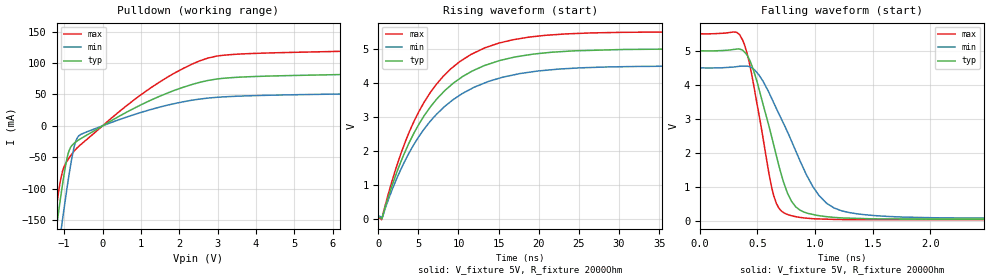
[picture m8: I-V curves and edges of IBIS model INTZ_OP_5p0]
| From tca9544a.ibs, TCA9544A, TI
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|   Model
[Model]   INTZ_OP_5p0
Model_type   Open_drain
Polarity   Non-Inverting
Vmeas = 2.5
Vref = 5
Cref = 1pF
Rref = 2000
|   typ   min   max
C_comp   1.601pF   1.487pF   1.862pF
[Voltage Range]   5   4.5   5.5
[Temperature Range]   27   125   -40
[Pullup Reference]   5   4.5   5.5
[Pulldown Reference]   -0   -0   -0
[Power Clamp Reference]   5   4.5   5.5
[GND Clamp Reference]   -0   -0   -0
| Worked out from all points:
|   slope of the pulldown table from 0 to 0.75 V, typ, clamps not added: 29.2 ohm
|   falling waveform, V_fixture 5V, R_fixture 2000Ohm: 20-80 % time 234ps typ, 368ps min, 171ps max; typ from 5 V to 0.068 V
|   rising waveform, V_fixture 5V, R_fixture 2000Ohm: 20-80 % time 7.63ns typ, 8.08ns min, 7.26ns max; typ from 0.068 V to 5 V
[Pulldown]
|   Voltage   I(typ)   I(min)   I(max)
-5V       -2.025A    -2.08A     -1.991A
-1.61V    -353.8mA   -413.6mA   -316.9mA
-1.25V    -183.9mA   -243.3mA   -148.6mA
-1.085V   -110.6mA   -167.8mA   -83.22mA
-1.025V   -85.9mA    -141.2mA   -68.54mA
-875mV    -39.88mA   -78.44mA   -51.42mA
-740mV    -27.74mA   -33.39mA   -40.24mA
-620mV    -22.36mA   -15.97mA   -32.64mA
1.27V     41.23mA    26.19mA    61.07mA
2.74V     72.2mA     44.16mA    107.9mA
7.435V    84.91mA    53.7mA     123.1mA
9.985V    125mA      83.55mA    179.8mA
[Ramp]
R_load = 2000
|   typ   min   max
dV/dt_r   2.95938/7.62679e-09   2.64368/8.08593e-09   3.26962/7.25871e-09
dV/dt_f   2.9594/2.33624e-10   2.64369/3.68147e-10   3.26964/1.70673e-10
[Falling Waveform]
V_fixture = 5V
V_fixture_min = 4.5V
V_fixture_max = 5.5V
R_fixture = 2000Ohm
C_fixture = 0F
|   Time   V(typ)   V(min)   V(max)
0s        5V         4.5V       5.5V
373.1ps   5.011V     4.551V     5.3V
461.7ps   4.47V      4.474V     4.089V
607.5ps   2.687V     3.719V     1.254V
685.3ps   1.636V     3.156V     389.6mV
830.9ps   430.4mV    2.073V     139.8mV
1.033ns   168.9mV    760.6mV    72.68mV
1.193ns   110.9mV    356.8mV    56.02mV
3.18ns    68.08mV    94.31mV    52mV
100ns     67.67mV    93.83mV    50.6mV
[Rising Waveform]
V_fixture = 5V
V_fixture_min = 4.5V
V_fixture_max = 5.5V
R_fixture = 2000Ohm
C_fixture = 0F
|   Time   V(typ)   V(min)   V(max)
0s        67.67mV    93.83mV    50.6mV
448.6ps   20.09mV    53.71mV    2.403mV
2.057ns   1.211V     1.055V     1.382V
3.952ns   2.295V     1.993V     2.611V
5.662ns   3.018V     2.633V     3.416V
7.167ns   3.495V     3.059V     3.941V
11.54ns   4.332V     3.828V     4.84V
16.68ns   4.748V     4.231V     5.268V
32.43ns   4.991V     4.489V     5.494V
100ns     5V         4.5V       5.5V
